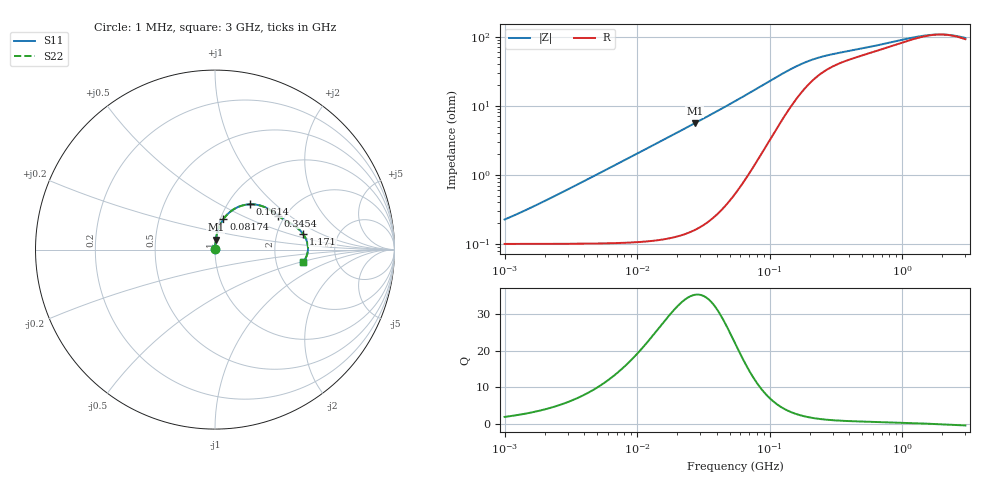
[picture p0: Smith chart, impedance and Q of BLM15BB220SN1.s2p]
! BLM15BB220SN1
# Hz S RI R 50
!Freq.(Hz) S11(Real) S11(Imag) S21(Real) S21(Imag) S12(Real) S12(Imag) S22(Real) S22(Imag)
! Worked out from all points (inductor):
!   401 points, 1 MHz to 3 GHz, reference 50 ohm
!   read as one part in series: L = 32.2 nH near 1.492 MHz
!   highest Q = 35.1 at 27.18 MHz (marker M1), where L = 32.6 nH
!   self-resonance near 1.991 GHz
!   S11 on the Smith chart (normalised r, x): 1 MHz: 1.00, +0.00; 81.74 MHz: 1.03, +0.36; 161.4 MHz: 1.26, +0.71; 345.4 MHz: 1.84, +0.83; 1.171 GHz: 2.80, +0.66; 3 GHz: 2.84, -0.53
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1000000  0.001 0.00202  0.999 -0.00202  0.999 -0.00202  0.001 0.00202
1173660  0.00101 0.00237  0.999 -0.00237  0.999 -0.00237  0.00101 0.00237
1649378  0.00101 0.00333  0.999 -0.00333  0.999 -0.00333  0.00101 0.00333
3823119  0.00107 0.00773  0.9989 -0.00773  0.9989 -0.00773  0.00107 0.00773
1.461624e7  0.00201 0.0296  0.998 -0.0296  0.998 -0.0296  0.00201 0.0296
2.718395e7  0.00467 0.0554  0.9953 -0.0554  0.9953 -0.0554  0.00467 0.0554
3.976269e7  0.00936 0.0817  0.9906 -0.0817  0.9906 -0.0817  0.00936 0.0817
5.477226e7  0.0184 0.1135  0.9816 -0.1135  0.9816 -0.1135  0.0184 0.1135
8.173662e7  0.0465 0.1692  0.9535 -0.1692  0.9535 -0.1692  0.0465 0.1692
9.593103e7  0.0679 0.1953  0.9321 -0.1953  0.9321 -0.1953  0.0679 0.1953
1.125904e8  0.098 0.2205  0.902 -0.2205  0.902 -0.2205  0.098 0.2205
1.348146e8  0.1425 0.2428  0.8575 -0.2428  0.8575 -0.2428  0.1425 0.2428
1.614254e8  0.1943 0.2524  0.8057 -0.2524  0.8057 -0.2524  0.1943 0.2524
2.094008e8  0.2657 0.2411  0.7343 -0.2411  0.7343 -0.2411  0.2657 0.2411
2.609752e8  0.3111 0.2184  0.6889 -0.2184  0.6889 -0.2184  0.3111 0.2184
3.453811e8  0.351 0.1899  0.649 -0.1899  0.649 -0.1899  0.351 0.1899
8.005644e8  0.4469 0.1297  0.5531 -0.1297  0.5531 -0.1297  0.4469 0.1297
1.171007e9  0.4895 0.0887  0.5105 -0.0887  0.5105 -0.0887  0.4895 0.0887
1.54974e9  0.5119 0.0458  0.4881 -0.0458  0.4881 -0.0458  0.5119 0.0458
1.931433e9  0.5182 0.00576  0.4818 -0.00576  0.4818 -0.00576  0.5182 0.00576
2.359433e9  0.5119 -0.0318  0.4881 0.0318  0.4881 0.0318  0.5119 -0.0318
3e9  0.4886 -0.0711  0.5114 0.0711  0.5114 0.0711  0.4886 -0.0711
